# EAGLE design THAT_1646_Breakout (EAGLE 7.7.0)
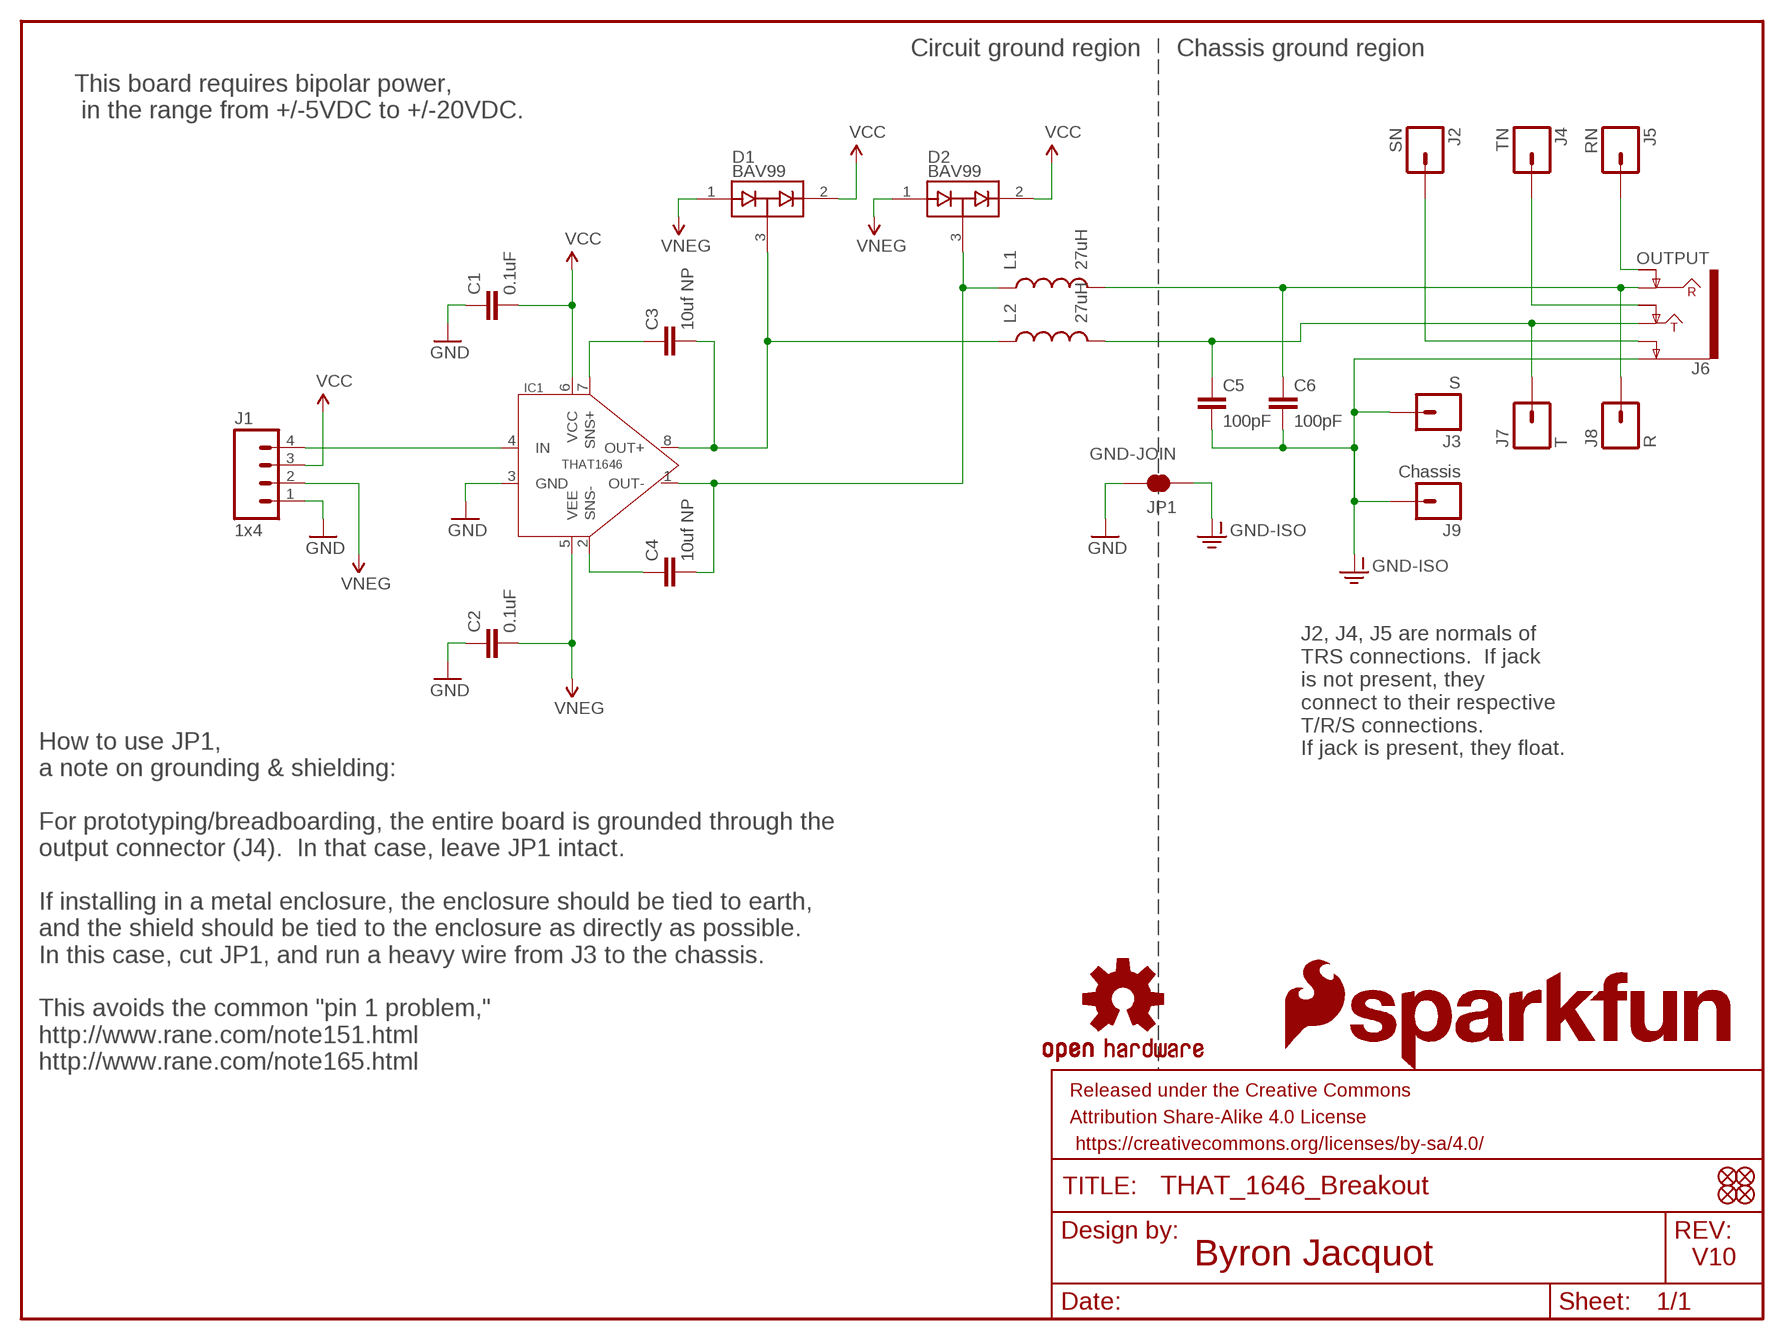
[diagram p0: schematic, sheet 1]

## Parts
C1  0.1uF  0.1UF-25V-5%(0603)  [0603-CAP]
C2  0.1uF  0.1UF-25V-5%(0603)  [0603-CAP]
C3  10uf NP  PANA-EEE-1EA100NP  [PANASONIC_D]
C4  10uf NP  PANA-EEE-1EA100NP  [PANASONIC_D]
C5  100pF  100PF-50V-5%(0603)  [0603-CAP]
C6  100pF  100PF-50V-5%(0603)  [0603-CAP]
D1  BAV99  [SOT23-3]
D2  BAV99  [SOT23-3]
FD1  FIDUCIALUFIDUCIAL  [MICRO-FIDUCIAL]
FD2  FIDUCIALUFIDUCIAL  [MICRO-FIDUCIAL]
FD3  FIDUCIALUFIDUCIAL  [MICRO-FIDUCIAL]
FD4  FIDUCIALUFIDUCIAL  [MICRO-FIDUCIAL]
FRAME1  FRAME-LETTER  [CREATIVE_COMMONS]
IC1  THAT1646  [SO08]
J1  1x4  M04NO_SILK_ALL_ROUND  [1X04_NO_SILK_ALL_ROUND]
J2  SN  M01PTH_NO_SILK_YES_STOP  [1X01_NO_SILK]
J3  S  M01PTH_NO_SILK_YES_STOP  [1X01_NO_SILK]
J4  TN  M01PTH_NO_SILK_YES_STOP  [1X01_NO_SILK]
J5  RN  M01PTH_NO_SILK_YES_STOP  [1X01_NO_SILK]
J6  OUTPUT  AUDIO_JACK_TRS_0.25"_PTH_RA  [AUDIO_JACK_0.25"_TRS_PTH_RA]
J7  T  M01PTH_NO_SILK_YES_STOP  [1X01_NO_SILK]
J8  R  M01PTH_NO_SILK_YES_STOP  [1X01_NO_SILK]
J9  Chassis  M01PTH_NO_SILK_YES_STOP  [1X01_NO_SILK]
JP1  GND-JOIN  JUMPER-PAD-2-NC_BY_TRACE  [PAD-JUMPER-2-NC_BY_TRACE_YES_SILK]
L1  27uH  INDUCTOR0603  [0603]
L2  27uH  INDUCTOR0603  [0603]
LOGO1  OSHW-LOGOS  [OSHW-LOGO-S]
LOGO2  OSHW-LOGOS  [OSHW-LOGO-S]
LOGO4  SFE_LOGO_FLAME.2_INCH  [SFE_LOGO_FLAME_.2]
LOGO5  SFE_LOGO_NAME.1_INCH  [SFE_LOGO_NAME_.1]

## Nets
GND: C1.1 C2.1 IC1.3(GND) J1.1 JP1.2
GND-ISO: C5.2 C6.2 J3.1 J6.SLEEVE(EARTH) J9.1 JP1.1
N$1: J5.1 J6.RING-NORM
N$2: J4.1 J6.TIP-NORM
N$3: J2.1 J6.SLEEVE-NORM(EARTH-NORM)
N$8: C5.1 J6.TIP J7.1 L2.2
N$9: C6.1 J6.RING J8.1 L1.2
N$10: C3.- D1.3(COM) IC1.8(OUT+) L2.1
N$11: C4.- D2.3(COM) IC1.1(OUT-) L1.1
N$13: C4.+ IC1.2(SNS-)
N$14: C3.+ IC1.7(SNS+)
N$16: IC1.4(IN) J1.4
VCC: C1.2 D1.2(C2) D2.2(C2) IC1.6(VCC) J1.3
VNEG: C2.2 D1.1(A1) D2.1(A1) IC1.5(VEE) J1.2

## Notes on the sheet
- Circuit ground region | Chassis ground region
- This board requires bipolar power,
   in the range from +/-5VDC to +/-20VDC.
- J2, J4, J5 are normals of 
  TRS connections.  If jack 
  is not present, they 
  connect to their respective 
  T/R/S connections.  
  If jack is present, they float.
- How to use JP1,
  a note on grounding & shielding:
  
  For prototyping/breadboarding, the entire board is grounded through the 
  output connector (J4).  In that case, leave JP1 intact.
  
  If installing in a metal enclosure, the enclosure should be tied to earth, 
  and the shield should be tied to the enclosure as directly as possible.  
  In this case, cut JP1, and run a heavy wire from J3 to the chassis.
  
  This avoids the common "pin 1 problem," 
  http://www.rane.com/note151.html
  http://www.rane.com/note165.html
- Byron Jacquot | V10

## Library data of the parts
C1 C2 = SparkFun-Capacitors:0.1UF-25V-5%(0603): CAP-08604; PROD_ID: CAP-08604
C3 C4 = that-ics:PANA-EEE-1EA100NP: Panasonic 10uf 25V nonpolar.; DK_PN: PCE4294TR-ND; MFR: Panasonic; MFR_PN: 1ea100np; PROD_ID: CAP-13474
C5 C6 = SparkFun-Capacitors:100PF-50V-5%(0603): CAP-07883; PROD_ID: CAP-07883
D1 D2 = SparkFun-DiscreteSemi:BAV99: Two small signal silicon diodes connected anode to cathode. Connections to all three nodes available. DIO-10647; PROD_ID: DIO-10647
FD1-FD4 = SparkFun-Aesthetics:FIDUCIAL: Fiducial Alignment Points
FRAME1 = SparkFun-Aesthetics:FRAME-LETTER: Schematic Frame
IC1 = that-ics:THAT1646: THAT Corporation 1646 OutSmarts Balanced line driver; PROD_ID: IC-13473
J1 = SparkFun-Connectors:M04: Header 4 Standard 4-pin 0.1" header. Use with straight break away headers (SKU : PRT-00116), right angle break away headers (PRT-00553), swiss pins (PRT-00743), machine pins (PRT-00117), and female headers (PRT-00115). Molex polarized connector foot print use with SKU : PRT-08231 with associated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; PROD_ID: CONN-09696
J2-J5 J7-J9 = SparkFun-Connectors:M01: Header 1
J6 = SparkFun-Connectors:AUDIO_JACK_TRS_0.25"_PTH_RA: Audio Jack, 1/4" TRS jack, horizontal, PTH, aka "Phono jack" Find the connector here: Audio Jack - 1/4" Stereo (right angle) (COM-11144) Datasheet Note, although the datasheet and physical part are slightly different, this footprint was proven to mate well on the Proto Pedal. This device is used on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; PROD_ID: CONN-12339; SF_ID: COM-11144
JP1 = SparkFun-Passives:JUMPER-PAD-2-NC_BY_TRACE
L1 L2 = SparkFun-Passives:INDUCTOR: Inductors; PROD_ID: NDUC-12579
LOGO1 LOGO2 = SparkFun-Aesthetics:OSHW-LOGO: Open Source Hardware Logo
LOGO4 = SparkFun-Aesthetics:SFE_LOGO_FLAME: SFE Logo, flame only
LOGO5 = SparkFun-Aesthetics:SFE_LOGO_NAME: SFE Logo, name only

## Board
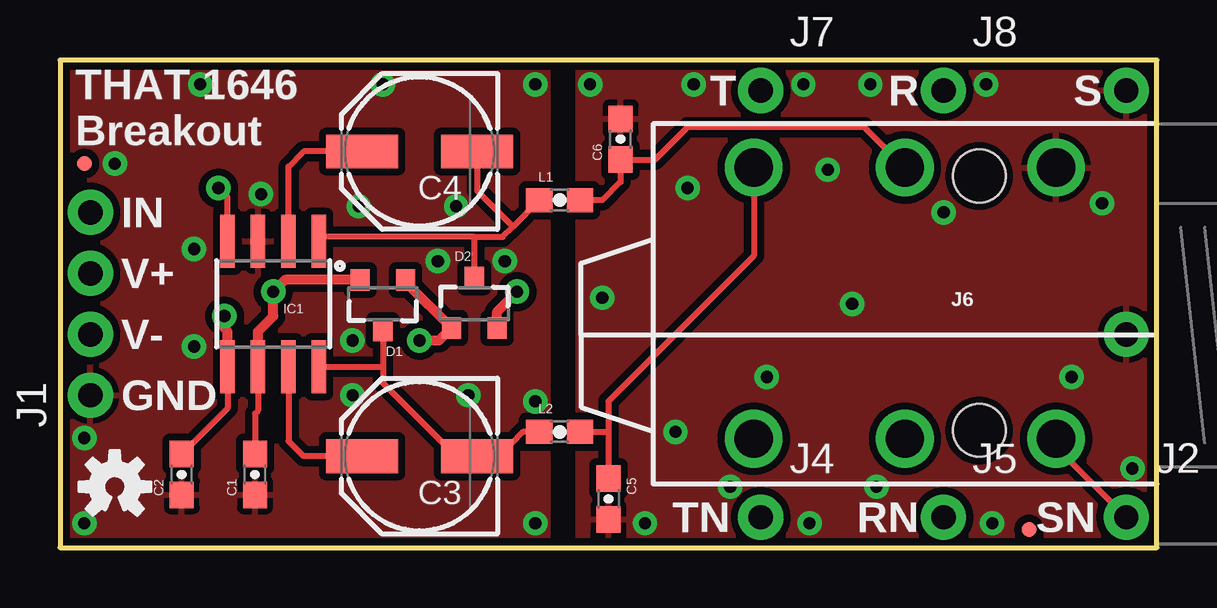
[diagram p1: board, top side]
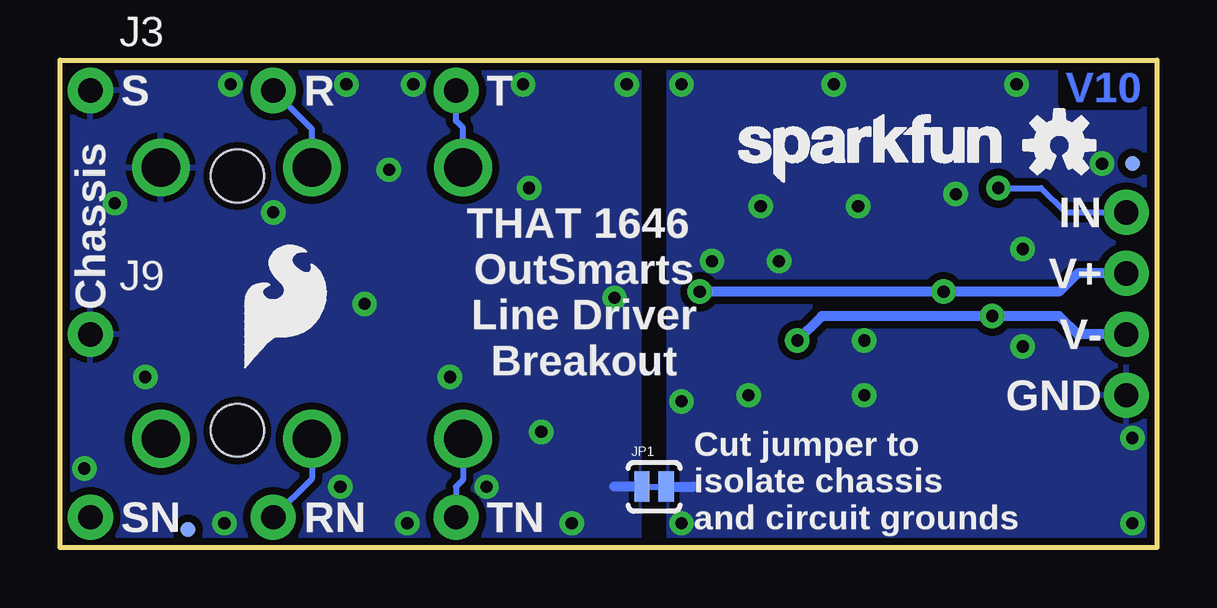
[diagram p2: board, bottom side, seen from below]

Size 45.72 x 20.32 mm. Coordinates in mm from the lower left corner, seen from the top.
Outline: 0,0 45.72,0 45.72,20.32 0,20.32 0,0
Copper layers (1*16): Top 0.035mm / dielectric 1.5mm / Bottom 0.035mm
Design rules "SparkFun-2-layer-STANDARD": minimum track width 10mil, minimum drill 20mil, track to track 10mil, track to pad 8mil, pad to pad 8mil, via to via 10mil, smd to smd 8mil, copper to edge 8mil, drill to drill 8mil, minimum pad ring 10mil, minimum via ring 10mil, stop-mask expansion 4mil, vias tented up to drill 25mil, thermal gap 10mil

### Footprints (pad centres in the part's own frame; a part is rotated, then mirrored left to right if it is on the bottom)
0603-CAP = smd 1.1 x 1: 1 -0.85,0; 2 0.85,0
PANASONIC_D = smd 3 x 1.4: + 2.4,0; - -2.4,0
SOT23-3 = smd 0.8 x 0.9: 1 -0.95,-1; 2 0.95,-1; 3 0,1.1
MICRO-FIDUCIAL = smd 0.635 x 0.635: 1 0,0
SO08 = smd 0.61 x 2.21: 1 -1.905,-2.616; 2 -0.635,-2.616; 3 0.635,-2.616; 4 1.905,-2.616; 5 1.905,2.616; 6 0.635,2.616; 7 -0.635,2.616; 8 -1.905,2.616
1X04_NO_SILK_ALL_ROUND = drill 1.016 pad 1.88: 1 0,0; 2 2.54,0; 3 5.08,0; 4 7.62,0
1X01_NO_SILK = drill 1.016 pad 1.88: 1 0,0
AUDIO_JACK_0.25"_TRS_PTH_RA = drill 1.6: RING 10.5,-6.95; RING-NORM 10.5,4.35; SLEEVE 4.2,-6.95; SLEEVE-NORM 4.2,4.35; TIP 16.8,-6.95; TIP-NORM 16.8,4.35 | hole 2.2: 7.4,4; 7.4,-6.6
PAD-JUMPER-2-NC_BY_TRACE_YES_SILK = smd 0.635 x 1.27: 1 -0.508,0; 2 0.508,0
0603 = smd 1.1 x 1: 1 -0.85,0; 2 0.85,0

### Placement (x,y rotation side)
C1  8.13,3.05 90 top
C2  5.08,3.05 90 top
C3  14.99,3.81 180 top
C4  14.99,16.51 180 top
C5  22.86,2.03 270 top
C6  23.37,17.02 90 top
D1  13.46,10.16 180 top
D2  17.27,10.16 0 top
FD1  1.02,16 0 bottom
FD2  40.39,0.76 0 bottom
FD3  1.02,16 0 top
FD4  40.39,0.76 0 top
FRAME1  not placed on the board
IC1  8.89,10.16 180 top
J1  1.27,6.35 90 top
J2  44.45,1.27 0 top
J3  44.45,19.05 0 bottom
J4  29.21,1.27 0 top
J5  36.83,1.27 0 top
J6  45.72,8.89 180 top
J7  29.21,19.05 0 top
J8  36.83,19.05 0 top
J9  44.45,8.89 0 bottom
JP1  20.95,2.54 0 bottom
L1  20.83,14.48 0 top
L2  20.83,4.83 0 top
LOGO1  2.29,2.54 0 top
LOGO2  4.06,16.76 0 bottom
LOGO4  38.35,7.24 0 bottom
LOGO5  17.91,14.73 0 bottom

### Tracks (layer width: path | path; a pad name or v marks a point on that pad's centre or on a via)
GND  (via drill 0.51)
  Bottom 0.406: JP1.2 19.3,2.54
  other vias: 1.02,1.02 5.59,8.38 5.59,12.45 1.02,4.57 2.29,16 5.84,19.3 19.81,19.3 18.54,11.94 15.75,11.94 12.19,8.64 12.19,6.35 17.02,6.35 19.81,6.1 19.81,1.02 8.38,14.73 12.45,14.22 16.51,14.22 13.46,19.3
  pour Top (isolate 0.305): 20.32,20.32 20.32,0 0,0 0,20.32
  pour Bottom (isolate 0.305): 0,20.32 0,0 20.32,0 20.32,20.32
GND-ISO  (via drill 0.51)
  Bottom 0.406: JP1.1 22.61,2.54
  other vias: 22.1,19.3 26.42,19.3 36.83,13.97 42.16,7.11 33.02,10.16 29.46,7.11 31.24,1.02 27.94,2.54 34.04,2.54 44.7,3.3 22.61,10.41 26.16,14.99 25.65,4.83 38.86,1.02 32,15.75 30.99,19.3 33.78,19.3 38.61,19.3 24.38,1.02 43.43,14.35
  pour Bottom (isolate 0.305): 21.59,0 21.59,20.32 45.72,20.32 45.72,0
  pour Top (isolate 0.305): 45.72,0 45.72,20.32 21.59,20.32 21.59,0
N$1
  Bottom 0.254: J6.RING-NORM 35.22,2.88 J5.1
N$2
  Bottom 0.254: J6.TIP-NORM 28.92,2.83 29.21,2.54 J4.1
N$3
  Top 0.254: J2.1 41.52,4.2 J6.SLEEVE-NORM
N$8
  Top 0.254: 22.86,4.83 22.86,6.1 28.92,12.16 J6.TIP | 22.86,4.83 C5.1 | L2.2 22.86,4.83
  Bottom 0.254: J6.TIP 28.92,17.49 29.21,17.78 J7.1
N$9
  Top 0.254: L1.2 22.61,14.48 23.37,15.24 C6.1 24.8,16.17 26.16,17.53 33.53,17.53 J6.RING
  Bottom 0.254: J6.RING 35.22,17.44 J8.1
N$10
  Top 0.254: IC1.8 13.46,7.54 | D1.3 13.46,7.54 | L2.1 19.3,4.83 18.8,4.32 17.89,4.32 C3.- 17.13,4.06 16.26,4.06 13.46,6.86 13.46,7.54
N$11
  Top 0.254: 17.27,12.95 10.97,12.95 IC1.1 | D2.3 17.27,12.95 | 18.88,13.38 18.45,12.95 17.27,12.95 | 18.88,13.38 L1.1 | C4.- 17.39,14.87 18.88,13.38
N$13
  Top 0.254: IC1.2 9.53,15.88 10.16,16.51 C4.+
N$14
  Top 0.254: IC1.7 9.53,4.45 10.16,3.81 C3.+
N$16  (via drill 0.51)
  Top 0.254: IC1.4 6.99,14.61 v6.6,14.99
  Bottom 0.254: v6.6,14.99 4.83,14.99 3.81,13.97 J1.4
VCC  (via drill 0.51)
  Top 0.254: IC1.6 8.26,5.71 8.13,5.59 C1.2
  Top 0.406: D2.2 18.22,9.84 v19.05,10.67 | IC1.6 8.26,9.02 8.89,9.65 v8.89,10.67 9.38,11.16 D1.2
  Bottom 0.406: J1.3 3.3,11.43 4.06,10.67 v8.89,10.67 v19.05,10.67
VNEG  (via drill 0.51)
  Top 0.254: D1.1 14.41,11.07 | IC1.5 6.99,5.8 C2.2
  Top 0.406: 14.41,11.07 D2.1 15.8,8.64 v14.99,8.64 | IC1.5 6.99,9.02 6.86,9.14 v6.86,9.65
  Bottom 0.406: J1.2 3.3,8.89 4.06,9.65 v6.86,9.65 13.97,9.65 v14.99,8.64

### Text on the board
Bottom: V10
tPlace: T | R | S | THAT 1646 / Breakout | IN | V+ | V- | GND | TN | RN | SN
bPlace: T | R | S | IN | V+ | THAT 1646 / OutSmarts / Line Driver / Breakout | Chassis | V- | GND | Cut jumper to / isolate chassis / and circuit grounds | TN | RN | SN
Measures: Drill 0.440" (11mm) hole to / accomodate TRS jack | All dimensions in inches
tDocu: Byron Jacquot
